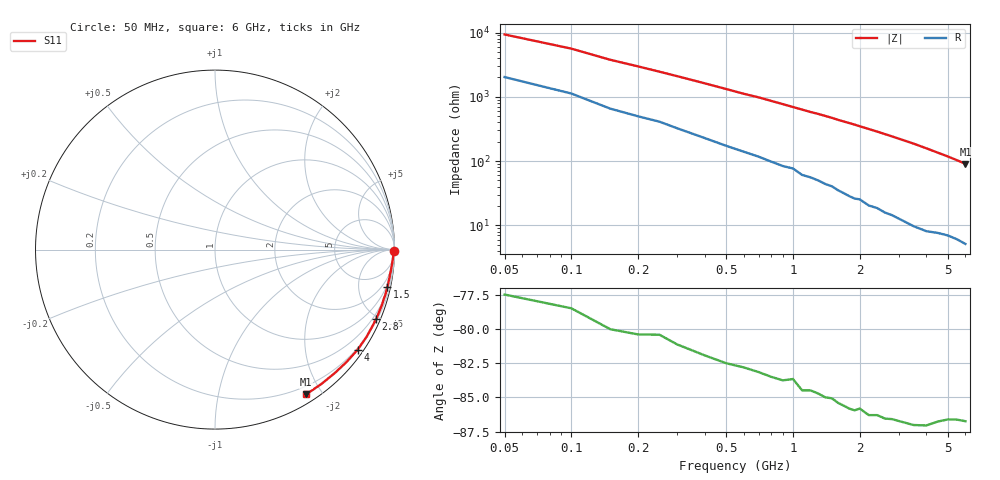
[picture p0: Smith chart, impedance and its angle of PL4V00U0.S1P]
! Infineon Technologies  Discrete & RF Semiconductors
! BAR 64-04W /-05W /-06W
! Si PIN Diode in SOT323
! VR = 4 V
! S-Parameters:  October  2008
# GHz  S  MA  R  50
!  f  S11
! GHz  MAG  ANG
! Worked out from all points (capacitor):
!   34 points, 50 MHz to 6 GHz, reference 50 ohm
!   read as one part to ground: C = 289 fF near 50 MHz
!   lowest |Z| = 90.5 ohm at 6 GHz (marker M1)
!   S11 on the Smith chart (normalised r, x): 50 MHz: open; 1.5 GHz: 0.81, -9.37; 2.8 GHz: 0.29, -4.83; 4 GHz: 0.16, -3.15; 6 GHz: 0.10, -1.81
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0.05  0.9977 -0.6
0.1  0.9964 -1.0
0.15  0.9954 -1.5
0.25  0.9932 -2.3
0.4  0.9914 -3.5
0.6  0.9888 -5.1
0.7  0.9879 -5.8
0.8  0.987 -6.6
0.9  0.986 -7.4
1  0.9842 -8.2
1.1  0.985 -9.0
1.2  0.9837 -9.8
1.3  0.9833 -10.5
1.5  0.9821 -12.1
1.6  0.9821 -13.0
1.9  0.9813 -15.4
2  0.9797 -16.3
2.2  0.9802 -18.0
2.4  0.9784 -19.7
2.6  0.9781 -21.5
2.8  0.9767 -23.3
3  0.9759 -25.2
3.5  0.9744 -29.9
4  0.9709 -35.1
4.5  0.964 -40.5
5  0.9584 -45.9
5.5  0.9548 -51.7
6  0.953 -57.8
